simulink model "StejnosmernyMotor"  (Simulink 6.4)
settings: Solver=ode45  StartTime=0.0  StopTime=10.0  MaxStep=1e-3  RelTol=1e-3

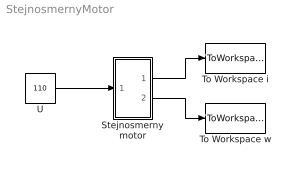
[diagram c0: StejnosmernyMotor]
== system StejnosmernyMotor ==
  Stejnosmerny motor : Subsystem
  To Workspace i : ToWorkspace  VariableName=i  SampleTime=-1  SaveFormat=Structure With Time
  To Workspace w : ToWorkspace  VariableName=w  SampleTime=-1  SaveFormat=Structure With Time
  U : Constant  Value=110  OutDataType=sfix(16)  ConRadixGroup=Use specified scaling  OutScaling=2^0  SampleTime=inf  FramePeriod=inf
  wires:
  U/1 -> Stejnosmerny motor/1(U)
  Stejnosmerny motor/1(" i") -> To Workspace i/1
  Stejnosmerny motor/2(w) -> To Workspace w/1

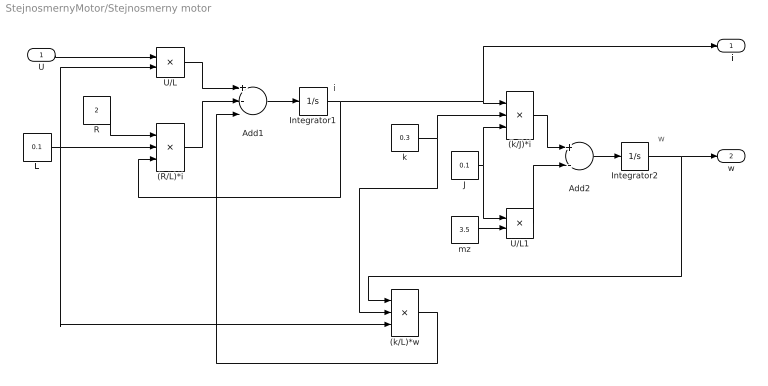
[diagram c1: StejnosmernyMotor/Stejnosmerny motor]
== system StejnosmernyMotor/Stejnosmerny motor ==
  note: i
  note: w
  U : Inport
  (R/L)*i : Product  Inputs=*/*  OutScaling=2^-10
  (k/J)*i : Product  Inputs=**/  OutScaling=2^-10
  (k/L)*w : Product  Inputs=**/  OutScaling=2^-10
  Add1 : Sum  Inputs=+--  OutScaling=2^-10
  Add2 : Sum  Inputs=+-  OutScaling=2^-10
  Integrator1 : Integrator
  Integrator2 : Integrator
  J : Constant  Value=0.1  OutDataType=sfix(16)  ConRadixGroup=Use specified scaling  OutScaling=2^0  SampleTime=inf  FramePeriod=inf
  L : Constant  Value=0.1  OutDataType=sfix(16)  ConRadixGroup=Use specified scaling  OutScaling=2^0  SampleTime=inf  FramePeriod=inf
  R : Constant  Value=2  OutDataType=sfix(16)  ConRadixGroup=Use specified scaling  OutScaling=2^0  SampleTime=inf  FramePeriod=inf
  U/L : Product  Inputs=*/  OutScaling=2^-10
  U/L1 : Product  Inputs=/*  OutScaling=2^-10
  k : Constant  Value=0.3  OutDataType=sfix(16)  ConRadixGroup=Use specified scaling  OutScaling=2^0  SampleTime=inf  FramePeriod=inf
  mz : Constant  Value=3.5  OutDataType=sfix(16)  ConRadixGroup=Use specified scaling  OutScaling=2^0  SampleTime=inf  FramePeriod=inf
  " i" : Outport
  w : Outport  Port=2
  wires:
  U/1 -> U/L/1
  L/1 -> U/L/2, (R/L)*i/2, (k/L)*w/3
  Add1/1 -> Integrator1/1
  U/L/1 -> Add1/1
  R/1 -> (R/L)*i/1
  Integrator1/1 -> (k/J)*i/1, " i"/1, (R/L)*i/3
  (R/L)*i/1 -> Add1/2
  Integrator2/1 -> (k/L)*w/1, w/1
  k/1 -> (k/J)*i/2, (k/L)*w/2
  Add2/1 -> Integrator2/1
  (k/J)*i/1 -> Add2/1
  J/1 -> (k/J)*i/3, U/L1/1
  U/L1/1 -> Add2/2
  mz/1 -> U/L1/2
  (k/L)*w/1 -> Add1/3
